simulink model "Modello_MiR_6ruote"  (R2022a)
settings: Solver=VariableStepAuto  StartTime=0.0  StopTime=time_v(end,1)  RelTol=1e-3
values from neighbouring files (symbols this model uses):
  a = 0.250    (= 0.25)    [Modello_MiR_6ruote_script.m]    (also in Modello_MiR_2ruote_script.m; Modello_MiR_6ruote_validato_script.m; Modello_MiR_UR_script.m)
  Att_C = 0.005    [Modello_MiR_6ruote_script.m]
  b = 0.1875    [Modello_MiR_6ruote_script.m]    (also in Modello_MiR_2ruote_script.m; Modello_MiR_6ruote_validato_script.m; Modello_MiR_UR_script.m)
  b_caster = 0.07    [Modello_MiR_6ruote_script.m]    (also in Modello_MiR_2ruote_script.m; Modello_MiR_6ruote_validato_script.m; Modello_MiR_UR_script.m)
  bd = 0.205    [Modello_MiR_6ruote_script.m]    (also in Modello_MiR_2ruote_script.m; Modello_MiR_6ruote_validato_script.m; Modello_MiR_UR_script.m)
  F23fun = @(u) (mv*9.801/4)-u(7)    [Modello_MiR_6ruote_script.m]    (also in Modello_MiR_6ruote_validato_script.m = @(u) (mv*9.801/4)-(mv*h*u(5)+(mv*9.801/4)*(2*a-b_caster*(cos)
  F43fun = @(u) (1/(2*bd))*(mv*u(6)*h+u(7)*(2*bd-b_caster*(sin(u(3))+sin(u(4))))+u(8)*(2*bd-b_caster*(sin(u(1))+sin(u(2)))))    [Modello_MiR_6ruote_script.m]    (also in Modello_MiR_6ruote_validato_script.m = @(u) (1/(2*bd))*(mv*u(6)*h+((mv*h*u(5)+(mv*9.801/4)*(2*a-b_c)
  F63fun = @(u) (mv*h*u(5)+(mv*9.801/4)*(2*a-b_caster*(cos(u(1))+cos(u(2)))))/(4*a-b_caster*(cos(u(1))+cos(u(2)))+b_caster*(cos(u(3))+cos(u(4))))    [Modello_MiR_6ruote_script.m]    (also in Modello_MiR_6ruote_validato_script.m)
  fm_fun = @(u) (u <= -am2 | u >= am2)*0 + (u > -am2 && u <= -am1)*(- u * Mza/(am2 -am1) - Mza * am2/(am2 -am1)) +           + (u > -am1 && u <= am1)*(Mza*u/ am1) + (u > am1 && u < am2)*(Mza * u/(am1 -am2) - Mza * am2/(am1 - am2))    [Modello_MiR_6ruote_script.m]    (also in Modello_MiR_6ruote_validato_script.m = @(u) (u <= -am2 || u >= am2) * 0 + (u > -am2 && u <= -am1) *; Modello_MiR_UR_script.m = @(u) (u <= -am2 || u >= am2) * 0 + (u > -am2 && u <= -am1) *)
  Icw_1 = 1/2 * mcw * rc^2    (= 0.002004225735)    [Modello_MiR_6ruote_script.m]    (also in Modello_MiR_2ruote_script.m; Modello_MiR_6ruote_validato_script.m; Modello_MiR_UR_script.m)
  Icw_2 = 1/12 * mcw * ec^2 + 1/4 * mcw * rc^2    (= 0.00104098243873)    [Modello_MiR_6ruote_script.m]    (also in Modello_MiR_2ruote_script.m; Modello_MiR_6ruote_validato_script.m; Modello_MiR_UR_script.m)
  Idw_1 = 1/2 * mdw * rd^2    (= 0.00551836278784)    [Modello_MiR_6ruote_script.m]    (also in Modello_MiR_2ruote_script.m; Transfer_Function_Gol_Gcl.m = Inertia_vect(jj,1); Modello_MiR_6ruote_validato_script.m; Modello_MiR_UR_script.m)
  iMax = 20.7*1.1    (= 22.77)    [Modello_MiR_6ruote_script.m]    (also in Modello_MiR_2ruote_script.m; Modello_MiR_6ruote_validato_script.m; Modello_MiR_UR_script.m)
  Iv = mv * (l^2 + w^2)  / 12    (= 6.75343333333)    [Modello_MiR_6ruote_script.m]    (also in Modello_MiR_2ruote_script.m; Modello_MiR_6ruote_validato_script.m = 8.95033333333; Modello_MiR_UR_script.m)
  Kc = 0.15    [Modello_MiR_6ruote_script.m]    (also in Modello_MiR_2ruote_script.m; Modello_MiR_6ruote_validato_script.m; Modello_MiR_UR_script.m)
  Ki_i = 1    [Modello_MiR_6ruote_script.m]    (also in Modello_MiR_2ruote_script.m; Modello_MiR_6ruote_validato_script.m; Modello_MiR_UR_script.m)
  Ki_v = 1    [Modello_MiR_6ruote_script.m]    (also in Modello_MiR_2ruote_script.m; Modello_MiR_6ruote_validato_script.m; Modello_MiR_UR_script.m)
  kk = 0.00005    (= 5e-05)    [Modello_MiR_6ruote_script.m]    (also in Modello_MiR_2ruote_script.m; Modello_MiR_6ruote_validato_script.m; Modello_MiR_UR_script.m)
  Kp_i = 5    [Modello_MiR_6ruote_script.m]    (also in Modello_MiR_2ruote_script.m; Modello_MiR_6ruote_validato_script.m; Modello_MiR_UR_script.m)
  Kp_v = 5    [Modello_MiR_6ruote_script.m]    (also in Modello_MiR_2ruote_script.m; Modello_MiR_6ruote_validato_script.m; Modello_MiR_UR_script.m)
  kv = 1.5e-6    (= 1.5e-06)    [Modello_MiR_6ruote_script.m]    (also in Modello_MiR_2ruote_script.m; Modello_MiR_6ruote_validato_script.m; Modello_MiR_UR_script.m)
  L = R * tauE    (= 0.00181134822805)    [Modello_MiR_6ruote_script.m]    (also in Modello_MiR_2ruote_script.m; Modello_MiR_6ruote_validato_script.m; Modello_MiR_UR_script.m)
  mcw = rc^2 * pi * ec * rhopoliu + 1    (= 1.02616357632)    [Modello_MiR_6ruote_script.m]    (also in Modello_MiR_2ruote_script.m; Modello_MiR_6ruote_validato_script.m; Modello_MiR_UR_script.m)
  mv = 83    [Modello_MiR_6ruote_script.m]    (also in Modello_MiR_2ruote_script.m; Modello_MiR_6ruote_validato_script.m = 110; Modello_MiR_UR_script.m)
  Psi_start = pi/2    (= 1.57079632679)    [Modello_MiR_6ruote_script.m]    (also in Modello_MiR_6ruote_validato_script.m = psi_mir(1,1); Modello_MiR_UR_script.m = psi_mir(1,1))
  R = velMax * TorqueMax / (iMax)^2    (= 1.81134822805)    [Modello_MiR_6ruote_script.m]    (also in Modello_MiR_2ruote_script.m; Modello_MiR_6ruote_validato_script.m; Modello_MiR_UR_script.m)
  rap_rid = 10.167    [Modello_MiR_6ruote_script.m]    (also in Modello_MiR_2ruote_script.m; Modello_MiR_6ruote_validato_script.m; Modello_MiR_UR_script.m)
  rc = 0.125/2    (= 0.0625)    [Modello_MiR_6ruote_script.m]    (also in Modello_MiR_2ruote_script.m; Modello_MiR_6ruote_validato_script.m; Modello_MiR_UR_script.m)
  rd = 0.1    [Modello_MiR_6ruote_script.m]    (also in Modello_MiR_2ruote_script.m; Modello_MiR_6ruote_validato_script.m; Modello_MiR_UR_script.m)
  Sx = spline(x ,fl_fun(x),zx)    [Modello_MiR_6ruote_script.m]
  Sy = spline(x ,ft_fun(x),zy)    [Modello_MiR_6ruote_script.m]
  VaMax = Kc * velMax    (= 41.2443991527)    [Modello_MiR_6ruote_script.m]    (also in Modello_MiR_2ruote_script.m; Modello_MiR_6ruote_validato_script.m; Modello_MiR_UR_script.m)
  X_start = input('Inserire coordinata x iniziale')    [Modello_MiR_6ruote_script.m]    (also in Modello_MiR_2ruote_script.m; Modello_MiR_6ruote_validato_script.m = traj(1,1); Modello_MiR_UR_script.m = traj(1,1))
  Y_start = input('Inserire coordinata y iniziale')    [Modello_MiR_6ruote_script.m]    (also in Modello_MiR_2ruote_script.m; Modello_MiR_6ruote_validato_script.m = traj(1,2); Modello_MiR_UR_script.m = traj(1,2))
  zx = linspace(inferior,superi,10001)    [Modello_MiR_6ruote_script.m]
  zy = linspace(inferior,superi,10001)    [Modello_MiR_6ruote_script.m]
libraries: slpidlib x4
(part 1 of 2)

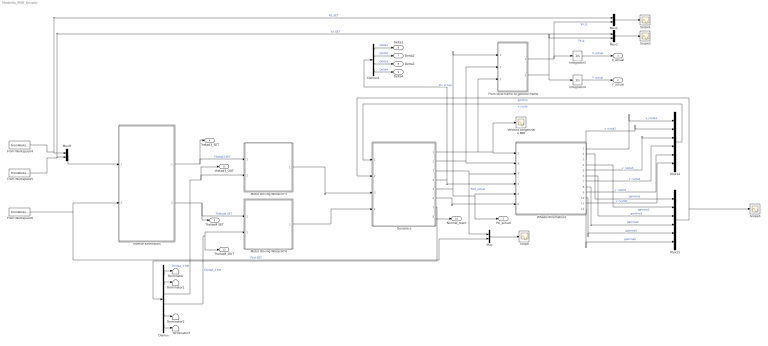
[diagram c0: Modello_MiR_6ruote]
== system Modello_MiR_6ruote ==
  " Wheels Kinematics1" : Subsystem
  Demux : Demux  Outputs=6
  Demux1 : Demux
  Dynamics : Subsystem
  From Workspace4 : FromWorkspace  VariableName=[time_v Xd_set]
  From Workspace5 : FromWorkspace  VariableName=[time_v Yd_set]
  From Workspace6 : FromWorkspace  VariableName=[ time_v psid_set]
  From local frame to general frame : Subsystem
  Integrator3 : Integrator  InitialCondition=X_start
  Integrator4 : Integrator  InitialCondition=Y_start
  Inverse Kinematics : Subsystem
  Motor Driving Wheel N°3 : Subsystem
  Motor Driving Wheel N°4 : Subsystem
  Mux{,1..2,9} (4 alike) : Mux  Inputs=2
  Mux14 : Mux  Inputs=6
  Mux15 : Mux  Inputs=6
  Scope{,1..3} (4 alike) : Scope
  Terminator{,1..3} (4 alike) : Terminator
  Velocità tangenziale MIR : Scope
  Psi_actual : Outport
  Y_actual : Outport  Port=2
  X_actual : Outport  Port=3
  Thetad3_SET : Outport  Port=4
  Thetad4 SET : Outport  Port=5
  Delta1 : Outport  Port=6
  Delta2 : Outport  Port=7
  Delta3 : Outport  Port=8
  Delta4 : Outport  Port=9
  Normal_react : Outport  Port=10
  thetad3_OUT : Outport  Port=11
  Thetad4_OUT : Outport  Port=12
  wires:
  From local frame to general frame/2(Vy_g) -> Mux2/2, Integrator4/1  "Vy_g"
  Mux2/1 -> Scope2/1
  Dynamics/6(Phid) -> " Wheels Kinematics1"/6(Phid)
  " Wheels Kinematics1"/9(v_ruota5) -> Mux14/5  "v_ruota5"
  " Wheels Kinematics1"/4(gamma2) -> Mux15/2  "gamma2"
  " Wheels Kinematics1"/11(v_ruota6) -> Mux14/6  "v_ruota6"
  " Wheels Kinematics1"/12(gamma6) -> Mux15/6  "gamma6"
  " Wheels Kinematics1"/10(gamma5) -> Mux15/5  "gamma5"
  " Wheels Kinematics1"/8(gamma4) -> Mux15/4  "gamma4"
  " Wheels Kinematics1"/3(v_ruota2) -> Mux14/2  "v_ruota2"
  Dynamics/7(Thetad) -> Demux/1
  Motor Driving Wheel N°3/1(Cm_L) -> Dynamics/3(Cm3)
  From Workspace6/1 -> Mux/2, Inverse Kinematics/2(PsiDotSet)  "Psid_SET"
  Mux/1 -> Scope/1
  Dynamics/4(Delta) -> " Wheels Kinematics1"/4(Delta), Demux1/1
  Dynamics/5(Psi) -> From local frame to general frame/1(Psi), " Wheels Kinematics1"/5(Psi), Psi_actual/1  "Psi_actual"
  " Wheels Kinematics1"/7(v_ruota4) -> Mux14/4  "v_ruota4"
  Demux/6 -> Terminator3/1
  Mux15/1 -> Scope3/1, Dynamics/2(gamma)  "gamma"
  " Wheels Kinematics1"/2(gamma1) -> Mux15/1  "gamma1"
  Demux/5 -> Terminator2/1
  Integrator4/1 -> Y_actual/1  "Y_actual"
  Mux9/1 -> Inverse Kinematics/1(vSet)
  Dynamics/1(xd) -> From local frame to general frame/3(Vx), " Wheels Kinematics1"/1(xd), Velocità tangenziale MIR/1
  " Wheels Kinematics1"/5(v_ruota3) -> Mux14/3  "v_ruota3"
  Dynamics/3(Psid) -> " Wheels Kinematics1"/3(Psid), Mux/1  "Psid_actual"
  " Wheels Kinematics1"/6(gamma3) -> Mux15/3  "gamma3"
  Integrator3/1 -> X_actual/1  "X_actual"
  Inverse Kinematics/2(ThetaDotR) -> Thetad4 SET/1, Motor Driving Wheel N°4/1(ThetadR_SET)  "Thetad4 SET"
  Demux/4 -> Thetad4_OUT/1, Motor Driving Wheel N°4/2(ThetadR_FB)  "Thetad_4 F/B"
  Demux/2 -> Terminator1/1
  From local frame to general frame/1(Vx_g) -> Mux1/2, Integrator3/1  "Vx_g"
  Mux14/1 -> Dynamics/1(v_ruote)  "v_ruote"
  Dynamics/2(yd) -> From local frame to general frame/2(Vy), " Wheels Kinematics1"/2(yd)
  Demux/1 -> Terminator/1
  " Wheels Kinematics1"/1(v_ruota1) -> Mux14/1  "v_ruota1"
  Inverse Kinematics/1(ThetaDotL) -> Thetad3_SET/1, Motor Driving Wheel N°3/1(ThetadL_SET)  "Thetad3 SET"
  Mux1/1 -> Scope1/1
  From Workspace5/1 -> Mux2/1, Mux9/2  "Yd_SET"
  Motor Driving Wheel N°4/1(Cm_R) -> Dynamics/4(Cm4)
  Demux/3 -> thetad3_OUT/1, Motor Driving Wheel N°3/2(ThetadL_FB)  "Thetad_3 F/B"
  From Workspace4/1 -> Mux1/1, Mux9/1  "Xd_SET"
  Demux1/1 -> Delta1/1  "Delta1"
  Demux1/2 -> Delta2/1  "Delta2"
  Demux1/3 -> Delta3/1  "Delta3"
  Demux1/4 -> Delta4/1  "Delta4"
  Dynamics/8(Normal_react) -> Normal_react/1

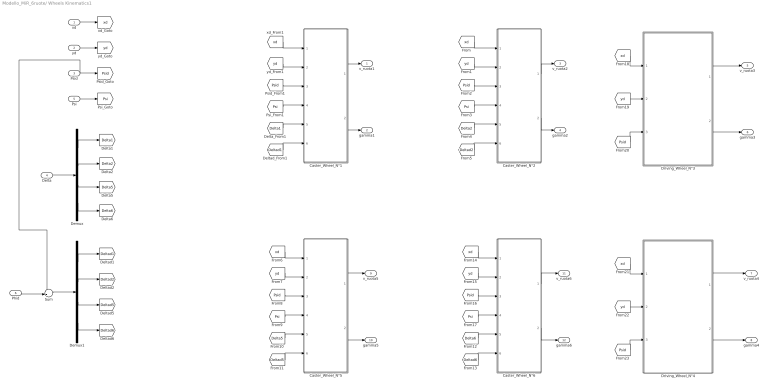
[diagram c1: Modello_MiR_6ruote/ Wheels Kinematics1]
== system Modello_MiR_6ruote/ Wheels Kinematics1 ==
  xd : Inport
  yd : Inport  Port=2
  Psid : Inport  Port=3
  Delta : Inport  Port=4
  Psi : Inport  Port=5
  Phid : Inport  Port=6
  Caster_Wheel_N°1 : Subsystem
  Caster_Wheel_N°2 : Subsystem
  Caster_Wheel_N°5 : Subsystem
  Caster_Wheel_N°6 : Subsystem
  Demux : Demux
  Demux1 : Demux
  Driving_Wheel_N°3 : Subsystem
  Driving_Wheel_N°4 : Subsystem
  Sum : Sum  Inputs=-+|
  v_ruota1 : Outport  PortDimensions=1
  gamma1 : Outport  Port=2  PortDimensions=1
  v_ruota2 : Outport  Port=3  PortDimensions=1
  gamma2 : Outport  Port=4  PortDimensions=1
  v_ruota3 : Outport  Port=5  PortDimensions=1
  gamma3 : Outport  Port=6  PortDimensions=1
  v_ruota4 : Outport  Port=7  PortDimensions=1
  gamma4 : Outport  Port=8  PortDimensions=1
  v_ruota5 : Outport  Port=9  PortDimensions=1
  gamma5 : Outport  Port=10  PortDimensions=1
  v_ruota6 : Outport  Port=11  PortDimensions=1
  gamma6 : Outport  Port=12  PortDimensions=1
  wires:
  xd/1 -> [xd]
  yd/1 -> [yd]
  Psid/1 -> [Psid], Sum/1
  Delta/1 -> Demux/1
  Demux/1 -> [Delta1]
  Demux/2 -> [Delta2]
  Demux/3 -> [Delta5]
  Demux/4 -> [Delta6]
  Psi/1 -> [Psi]
  Phid/1 -> Sum/2
  Demux1/1 -> [Deltad1]
  Demux1/2 -> [Deltad2]
  Demux1/3 -> [Deltad5]
  Demux1/4 -> [Deltad6]
  [xd] -> Caster_Wheel_N°1/1(xd_From1)
  [yd] -> Caster_Wheel_N°1/2(yd_From1)
  [Psid] -> Caster_Wheel_N°1/3(Psid_From1)
  [Psi] -> Caster_Wheel_N°1/4(Psi_From1)
  [Delta1] -> Caster_Wheel_N°1/5(Delta_From1)
  [Deltad1] -> Caster_Wheel_N°1/6(Deltad_From1)
  Caster_Wheel_N°1/1(v_ruota1) -> v_ruota1/1
  Caster_Wheel_N°1/2(gamma1) -> gamma1/1
  [yd] -> Caster_Wheel_N°2/2(yd_From1)
  [Psi] -> Caster_Wheel_N°2/4(Psi_From1)
  [Psid] -> Caster_Wheel_N°2/3(Psid_From1)
  [xd] -> Caster_Wheel_N°2/1(xd_From1)
  [Deltad2] -> Caster_Wheel_N°2/6(Deltad_From2)
  Caster_Wheel_N°2/2(gamma2) -> gamma2/1
  [Delta2] -> Caster_Wheel_N°2/5(Delta_From2)
  Caster_Wheel_N°2/1(v_ruota2) -> v_ruota2/1
  [xd] -> Caster_Wheel_N°5/1(xd_From1)
  Caster_Wheel_N°5/2(gamma5) -> gamma5/1
  Caster_Wheel_N°5/1(v_ruota5) -> v_ruota5/1
  [Psid] -> Caster_Wheel_N°5/3(Psid_From1)
  [Deltad5] -> Caster_Wheel_N°5/6(Deltad_From5)
  [yd] -> Caster_Wheel_N°5/2(yd_From1)
  [Delta5] -> Caster_Wheel_N°5/5(Delta_From5)
  [Psi] -> Caster_Wheel_N°5/4(Psi_From1)
  Caster_Wheel_N°6/1(v_ruota6) -> v_ruota6/1
  [yd] -> Caster_Wheel_N°6/2(yd_From1)
  [Psid] -> Caster_Wheel_N°6/3(Psid_From1)
  [Psi] -> Caster_Wheel_N°6/4(Psi_From1)
  Caster_Wheel_N°6/2(gamma6) -> gamma6/1
  [xd] -> Caster_Wheel_N°6/1(xd_From1)
  [Delta6] -> Caster_Wheel_N°6/5(Delta_From6)
  [Deltad6] -> Caster_Wheel_N°6/6(Deltad_From6)
  [xd] -> Driving_Wheel_N°3/1(xd_From1)
  [yd] -> Driving_Wheel_N°3/2(yd_From1)
  [Psid] -> Driving_Wheel_N°3/3(Psid_From1)
  [xd] -> Driving_Wheel_N°4/1(xd_From1)
  [yd] -> Driving_Wheel_N°4/2(yd_From1)
  [Psid] -> Driving_Wheel_N°4/3(Psid_From1)
  Driving_Wheel_N°3/1(v_ruota3) -> v_ruota3/1
  Driving_Wheel_N°3/2(gamma3) -> gamma3/1
  Driving_Wheel_N°4/1(v_ruota4) -> v_ruota4/1
  Driving_Wheel_N°4/2(gamma4) -> gamma4/1
  Sum/1 -> Demux1/1

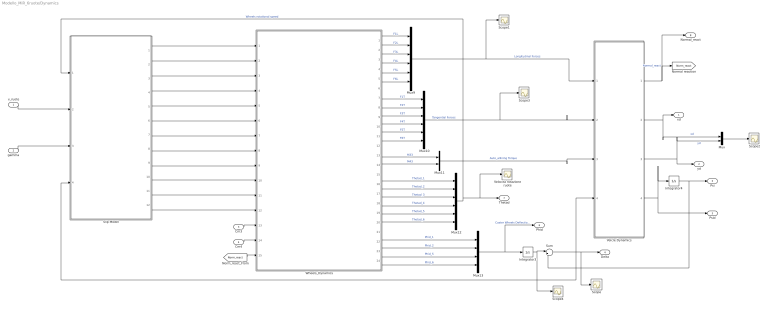
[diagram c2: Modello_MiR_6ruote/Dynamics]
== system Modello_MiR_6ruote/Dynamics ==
  v_ruote : Inport
  gamma : Inport  Port=2
  Cm3 : Inport  Port=3
  Cm4 : Inport  Port=4
  Integrator3 : Integrator  InitialCondition=Psi_start
  Integrator4 : Integrator  InitialCondition=Psi_start
  Mux : Mux  Inputs=2
  Mux10 : Mux  Inputs=6
  Mux11 : Mux  Inputs=2
  Mux12 : Mux  Inputs=6
  Mux13 : Mux
  Mux9 : Mux  Inputs=6
  Scope{,1..4} (5 alike) : Scope
  Slip Model : Subsystem
  Sum : Sum  Inputs=|+-
  Veicle Dynamics : Subsystem
  Velocità rotazione ruote : Scope
  Wheels_Dynamics : Subsystem
  xd : Outport
  yd : Outport  Port=2
  Psid : Outport  Port=3
  Delta : Outport  Port=4
  Psi : Outport  Port=5
  Phid : Outport  Port=6
  Thetad : Outport  Port=7
  Normal_react : Outport  Port=8
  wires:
  Wheels_Dynamics/14(M43) -> Mux11/2  "M43"
  Wheels_Dynamics/23(Phid_5) -> Mux13/3  "Phid_5"
  Wheels_Dynamics/8(F2T) -> Mux10/2  "F2T"
  Wheels_Dynamics/12(F6T) -> Mux10/6  "F6T"
  Wheels_Dynamics/19(Thetad_5) -> Mux12/5  "Thetad_5"
  Wheels_Dynamics/18(Thetad_4) -> Mux12/4  "Thetad_4"
  Slip Model/1(Sigma1) -> Wheels_Dynamics/1(Sigma1)
  Wheels_Dynamics/2(F2L) -> Mux9/2  "F2L"
  Wheels_Dynamics/4(F4L) -> Mux9/4  "F4L"
  Wheels_Dynamics/3(F3L) -> Mux9/3  "F3L"
  Veicle Dynamics/4(Psid) -> Psid/1, Integrator4/1
  Wheels_Dynamics/1(F1L) -> Mux9/1  "F1L"
  Slip Model/3(Sigma3) -> Wheels_Dynamics/3(Sigma3)
  Slip Model/11(alpha5) -> Wheels_Dynamics/11(alpha5)
  Wheels_Dynamics/5(F5L) -> Mux9/5  "F5L"
  Slip Model/9(alpha3) -> Wheels_Dynamics/9(alpha3)
  Wheels_Dynamics/16(Thetad_2) -> Mux12/2  "Thetad_2"
  Mux13/1 -> Integrator3/1, Phid/1  "Caster Wheels Deflection Velocity"
  Cm3/1 -> Wheels_Dynamics/13(Cm3)
  Mux11/1 -> Veicle Dynamics/3(M)  "Auto_allining Torque"
  Wheels_Dynamics/10(F4T) -> Mux10/4  "F4T"
  Wheels_Dynamics/13(M33) -> Mux11/1  "M33"
  Mux12/1 -> Slip Model/1(Thetad_ruote), Velocità rotazione ruote/1, Thetad/1  "Wheels rotational speed"
  Mux10/1 -> Scope3/1, Veicle Dynamics/2(FT)  "Tangential Forces"
  Slip Model/5(Sigma5) -> Wheels_Dynamics/5(Sigma5)
  Wheels_Dynamics/21(Phid_1) -> Mux13/1  "Phid_1"
  Wheels_Dynamics/6(F6L) -> Mux9/6  "F6L"
  Wheels_Dynamics/17(Thetad_3) -> Mux12/3  "Thetad_3"
  Wheels_Dynamics/15(Thetad_1) -> Mux12/1  "Thetad_1"
  Wheels_Dynamics/24(Phid_6) -> Mux13/4  "Phid_6"
  Wheels_Dynamics/11(F5T) -> Mux10/5  "F5T"
  Wheels_Dynamics/9(F3T) -> Mux10/3  "F3T"
  Wheels_Dynamics/7(F1T) -> Mux10/1  "F1T"
  Wheels_Dynamics/22(Phid_2) -> Mux13/2  "Phid_2"
  Veicle Dynamics/1(Normal_react) -> Normal_react/1, [Norm_react]  "Normal_react"
  Veicle Dynamics/2(xd) -> Mux/1, xd/1  "xd"
  Integrator3/1 -> Scope4/1, Sum/1
  Wheels_Dynamics/20(Thetad_6) -> Mux12/6  "Thetad_6"
  Slip Model/8(alpha2) -> Wheels_Dynamics/8(alpha2)
  Integrator4/1 -> Sum/2, Psi/1
  [Norm_react] -> Wheels_Dynamics/15(Normal_React)
  Veicle Dynamics/3(yd) -> Mux/2, yd/1  "yd"
  Mux9/1 -> Scope1/1, Veicle Dynamics/1(FL)  "Longitudinal Forces"
  Slip Model/4(Sigma4) -> Wheels_Dynamics/4(Sigma4)
  Slip Model/10(alpha4) -> Wheels_Dynamics/10(alpha4)
  Slip Model/12(alpha6) -> Wheels_Dynamics/12(alpha6)
  Slip Model/7(alpha1) -> Wheels_Dynamics/7(alpha1)
  Slip Model/2(Sigma2) -> Wheels_Dynamics/2(Sigma2)
  Slip Model/6(Sigma6) -> Wheels_Dynamics/6(Sigma6)
  v_ruote/1 -> Slip Model/2(v_ruote)
  gamma/1 -> Slip Model/3(gamma)
  Cm4/1 -> Wheels_Dynamics/14(Cm4)
  Mux/1 -> Scope2/1
  Sum/1 -> Slip Model/4(Delta), Scope/1, Delta/1, Veicle Dynamics/4(Delta)

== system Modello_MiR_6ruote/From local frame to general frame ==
  Psi : Inport
  Vy : Inport  Port=2
  Vx : Inport  Port=3
  Cos : Trigonometry  Operator=cos
  Product{,1..3} (4 alike) : Product
  Sin : Trigonometry
  Sum : Sum  Inputs=-+
  Sum1 : Sum  Inputs=|++
  Vx_g : Outport
  Vy_g : Outport  Port=2
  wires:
  Product/1 -> Sum/2
  Sin/1 -> Product2/2, Product1/2
  Product1/1 -> Sum/1
  Vx/1 -> Product2/1, Product/1
  Product2/1 -> Sum1/1
  Cos/1 -> Product3/1, Product/2
  Product3/1 -> Sum1/2
  Psi/1 -> Sin/1, Cos/1
  Vy/1 -> Product3/2, Product1/1
  Sum/1 -> Vx_g/1
  Sum1/1 -> Vy_g/1

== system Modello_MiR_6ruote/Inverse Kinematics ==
  vSet : Inport
  PsiDotSet : Inport  Port=2
  Demux : Demux  Outputs=2
  Integrator : Integrator  InitialCondition=Psi_start
  MATLAB Function : MATLAB Function  TreatAsAtomicUnit=on
  MATLAB Function1 : MATLAB Function  TreatAsAtomicUnit=on
  Scope1 : Scope
  Scope2 : Scope
  ThetaDotL : Outport
  ThetaDotR : Outport  Port=2
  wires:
  vSet/1 -> Demux/1
  Demux/1 -> MATLAB Function1/2(Xd_set), MATLAB Function/2(Xd_set)  "Xd_set"
  Demux/2 -> MATLAB Function1/3(Yd_set), MATLAB Function/3(Yd_set)  "Yd_set"
  PsiDotSet/1 -> MATLAB Function1/4(psid_set), MATLAB Function/4(psid_set), Integrator/1
  Integrator/1 -> MATLAB Function1/1(psi_set), MATLAB Function/1(psi_set)  "Psi_set"
  MATLAB Function/1(Thetad_DR_SET) -> Scope1/1, ThetaDotR/1
  MATLAB Function1/1(Thetad_DL_SET) -> Scope2/1, ThetaDotL/1

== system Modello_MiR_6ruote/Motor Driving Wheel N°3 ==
  ThetadL_SET : Inport
  ThetadL_FB : Inport  Port=2
  Gain : Gain  Gain=rap_rid
  Gain1 : Gain  Gain=rap_rid
  Subsystem : Subsystem
  Subsystem1 : Subsystem
  Cm_L : Outport  PortDimensions=1
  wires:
  Subsystem/1(VaRif) -> Subsystem1/1(VaRif)
  Subsystem1/2(iFB) -> Subsystem/3(iFB)
  ThetadL_SET/1 -> Gain1/1
  ThetadL_FB/1 -> Gain/1
  Subsystem1/1(Torque Cm) -> Cm_L/1
  Gain/1 -> Subsystem1/2(Thetad_FB), Subsystem/2(Thetad_FB)
  Gain1/1 -> Subsystem/1(Thetad_SET)

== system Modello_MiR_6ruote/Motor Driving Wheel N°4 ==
  ThetadR_SET : Inport
  ThetadR_FB : Inport  Port=2
  Gain : Gain  Gain=rap_rid
  Gain1 : Gain  Gain=rap_rid
  Subsystem : Subsystem
  Subsystem1 : Subsystem
  Cm_R : Outport  PortDimensions=1
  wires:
  Subsystem1/2(iFB) -> Subsystem/3(iFB)
  ThetadR_SET/1 -> Gain1/1
  Subsystem/1(VaRif) -> Subsystem1/1(VaRif)
  ThetadR_FB/1 -> Gain/1
  Subsystem1/1(Torque Cm) -> Cm_R/1
  Gain/1 -> Subsystem1/2(Thetad_FB), Subsystem/2(Thetad_FB)
  Gain1/1 -> Subsystem/1(Thetad_SET)

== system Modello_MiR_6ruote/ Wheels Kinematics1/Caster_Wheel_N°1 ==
  xd_From1 : Inport
  yd_From1 : Inport  Port=2
  Psid_From1 : Inport  Port=3
  Psi_From1 : Inport  Port=4
  Delta_From1 : Inport  Port=5
  Deltad_From1 : Inport  Port=6
  Interpreted MATLAB Function : MATLABFcn  MATLABFcn=(u(1)^2+u(2)^2)^0.5
  Interpreted MATLAB Function2 : MATLABFcn  MATLABFcn=asin(u(2)/((u(1)^2+u(2)^2)^0.5+1*(((u(1)^2+u(2)^2)^0.5)==0)))
  Mux : Mux  Inputs=6
  Mux1 : Mux  Inputs=2
  xd_ruota1 : MATLABFcn  MATLABFcn=(u(6)+u(3))*b_caster*sin(u(5))+u(1)-u(3)*b
  yd_ruota1 : MATLABFcn  MATLABFcn=-(u(6)+u(3))*b_caster*cos(u(5))+u(2)+u(3)*a
  v_ruota1 : Outport
  gamma1 : Outport  Port=2
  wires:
  Mux/1 -> xd_ruota1/1, yd_ruota1/1
  Mux1/1 -> Interpreted MATLAB Function/1, Interpreted MATLAB Function2/1
  yd_ruota1/1 -> Mux1/2  "yd_ruota1"
  yd_From1/1 -> Mux/2
  xd_ruota1/1 -> Mux1/1  "xd_ruota1"
  xd_From1/1 -> Mux/1
  Psid_From1/1 -> Mux/3
  Delta_From1/1 -> Mux/5
  Psi_From1/1 -> Mux/4
  Deltad_From1/1 -> Mux/6
  Interpreted MATLAB Function2/1 -> gamma1/1  "gamma1"
  Interpreted MATLAB Function/1 -> v_ruota1/1  "v_ruota1"

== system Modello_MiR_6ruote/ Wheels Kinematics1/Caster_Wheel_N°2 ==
  xd_From1 : Inport
  yd_From1 : Inport  Port=2
  Psid_From1 : Inport  Port=3
  Psi_From1 : Inport  Port=4
  Delta_From2 : Inport  Port=5
  Deltad_From2 : Inport  Port=6
  Interpreted MATLAB Function : MATLABFcn  MATLABFcn=(u(1)^2+u(2)^2)^0.5
  Interpreted MATLAB Function2 : MATLABFcn  MATLABFcn=asin(u(2)/((u(1)^2+u(2)^2)^0.5+1*(((u(1)^2+u(2)^2)^0.5)==0)))
  Mux : Mux  Inputs=6
  Mux1 : Mux  Inputs=2
  xd_ruota2 : MATLABFcn  MATLABFcn=(u(6)+u(3))*b_caster*sin(u(5))+u(1)+u(3)*b
  yd_ruota2 : MATLABFcn  MATLABFcn=-(u(6)+u(3))*b_caster*cos(u(5))+u(2)+u(3)*a
  v_ruota2 : Outport
  gamma2 : Outport  Port=2
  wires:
  Mux/1 -> xd_ruota2/1, yd_ruota2/1
  Mux1/1 -> Interpreted MATLAB Function/1, Interpreted MATLAB Function2/1
  yd_ruota2/1 -> Mux1/2  "yd_ruota2"
  yd_From1/1 -> Mux/2
  xd_ruota2/1 -> Mux1/1  "xd_ruota2"
  xd_From1/1 -> Mux/1
  Psid_From1/1 -> Mux/3
  Delta_From2/1 -> Mux/5
  Psi_From1/1 -> Mux/4
  Deltad_From2/1 -> Mux/6
  Interpreted MATLAB Function2/1 -> gamma2/1  "gamma2"
  Interpreted MATLAB Function/1 -> v_ruota2/1  "v_ruota2"

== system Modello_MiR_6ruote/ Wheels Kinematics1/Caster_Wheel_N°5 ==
  xd_From1 : Inport
  yd_From1 : Inport  Port=2
  Psid_From1 : Inport  Port=3
  Psi_From1 : Inport  Port=4
  Delta_From5 : Inport  Port=5
  Deltad_From5 : Inport  Port=6
  Interpreted MATLAB Function : MATLABFcn  MATLABFcn=(u(1)^2+u(2)^2)^0.5
  Interpreted MATLAB Function2 : MATLABFcn  MATLABFcn=asin(u(2)/((u(1)^2+u(2)^2)^0.5+1*(((u(1)^2+u(2)^2)^0.5)==0)))
  Mux : Mux  Inputs=6
  Mux1 : Mux  Inputs=2
  xd_ruota5 : MATLABFcn  MATLABFcn=(u(6)+u(3))*b_caster*sin(u(5))+u(1)-u(3)*a
  yd_ruota5 : MATLABFcn  MATLABFcn=-(u(6)+u(3))*b_caster*cos(u(5))+u(2)-u(3)*b
  v_ruota5 : Outport
  gamma5 : Outport  Port=2
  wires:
  Mux/1 -> xd_ruota5/1, yd_ruota5/1
  Mux1/1 -> Interpreted MATLAB Function/1, Interpreted MATLAB Function2/1
  yd_ruota5/1 -> Mux1/2  "yd_ruota5"
  yd_From1/1 -> Mux/2
  xd_ruota5/1 -> Mux1/1  "xd_ruota5"
  xd_From1/1 -> Mux/1
  Psid_From1/1 -> Mux/3
  Delta_From5/1 -> Mux/5
  Psi_From1/1 -> Mux/4
  Deltad_From5/1 -> Mux/6
  Interpreted MATLAB Function2/1 -> gamma5/1  "gamma5"
  Interpreted MATLAB Function/1 -> v_ruota5/1  "v_ruota5"

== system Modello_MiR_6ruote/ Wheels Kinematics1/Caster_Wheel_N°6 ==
  xd_From1 : Inport
  yd_From1 : Inport  Port=2
  Psid_From1 : Inport  Port=3
  Psi_From1 : Inport  Port=4
  Delta_From6 : Inport  Port=5
  Deltad_From6 : Inport  Port=6
  Interpreted MATLAB Function : MATLABFcn  MATLABFcn=(u(1)^2+u(2)^2)^0.5
  Interpreted MATLAB Function2 : MATLABFcn  MATLABFcn=asin(u(2)/((u(1)^2+u(2)^2)^0.5+1*(((u(1)^2+u(2)^2)^0.5)==0)))
  Mux : Mux  Inputs=6
  Mux1 : Mux  Inputs=2
  xd_ruota6 : MATLABFcn  MATLABFcn=(u(6)+u(3))*b_caster*sin(u(5))+u(1)+u(3)*b
  yd_ruota6 : MATLABFcn  MATLABFcn=-(u(6)+u(3))*b_caster*cos(u(5))+u(2)-u(3)*a
  v_ruota6 : Outport
  gamma6 : Outport  Port=2
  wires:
  Mux/1 -> xd_ruota6/1, yd_ruota6/1
  Mux1/1 -> Interpreted MATLAB Function/1, Interpreted MATLAB Function2/1
  yd_ruota6/1 -> Mux1/2  "yd_ruota6"
  yd_From1/1 -> Mux/2
  xd_ruota6/1 -> Mux1/1  "xd_ruota6"
  xd_From1/1 -> Mux/1
  Psid_From1/1 -> Mux/3
  Delta_From6/1 -> Mux/5
  Psi_From1/1 -> Mux/4
  Deltad_From6/1 -> Mux/6
  Interpreted MATLAB Function2/1 -> gamma6/1  "gamma6"
  Interpreted MATLAB Function/1 -> v_ruota6/1  "v_ruota6"

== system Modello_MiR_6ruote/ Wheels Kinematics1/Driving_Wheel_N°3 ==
  xd_From1 : Inport
  yd_From1 : Inport  Port=2
  Psid_From1 : Inport  Port=3
  Interpreted MATLAB Function : MATLABFcn  MATLABFcn=u(1) - u(3)*bd
  Interpreted MATLAB Function1 : MATLABFcn  MATLABFcn=u(2)
  Interpreted MATLAB Function3 : MATLABFcn  MATLABFcn=asin(u(2)/((u(1)^2+u(2)^2)^0.5+1*(((u(1)^2+u(2)^2)^0.5)==0)))
  Mux : Mux  Inputs=3
  Mux1 : Mux  Inputs=2
  Scope : Scope
  v_ruota3 : Outport
  gamma3 : Outport  Port=2
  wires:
  yd_From1/1 -> Mux/2
  xd_From1/1 -> Mux/1
  Psid_From1/1 -> Mux/3
  Mux/1 -> Interpreted MATLAB Function1/1, Interpreted MATLAB Function/1
  Interpreted MATLAB Function1/1 -> Mux1/2  "yd_ruota3"
  Interpreted MATLAB Function3/1 -> gamma3/1  "gamma3"
  Mux1/1 -> Interpreted MATLAB Function3/1
  Interpreted MATLAB Function/1 -> v_ruota3/1, Mux1/1, Scope/1  "v_ruota3"

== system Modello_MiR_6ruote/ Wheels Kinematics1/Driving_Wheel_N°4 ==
  xd_From1 : Inport
  yd_From1 : Inport  Port=2
  Psid_From1 : Inport  Port=3
  Interpreted MATLAB Function : MATLABFcn  MATLABFcn=u(1) + u(3)*bd
  Interpreted MATLAB Function1 : MATLABFcn  MATLABFcn=u(2)
  Interpreted MATLAB Function3 : MATLABFcn  MATLABFcn=asin(u(2)/((u(1)^2+u(2)^2)^0.5+1*(((u(1)^2+u(2)^2)^0.5)==0)))
  Mux : Mux  Inputs=3
  Mux1 : Mux  Inputs=2
  Scope : Scope
  v_ruota4 : Outport
  gamma4 : Outport  Port=2
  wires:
  yd_From1/1 -> Mux/2
  xd_From1/1 -> Mux/1
  Psid_From1/1 -> Mux/3
  Mux/1 -> Interpreted MATLAB Function1/1, Interpreted MATLAB Function/1
  Interpreted MATLAB Function1/1 -> Mux1/2  "yd_ruota4"
  Mux1/1 -> Interpreted MATLAB Function3/1
  Interpreted MATLAB Function/1 -> v_ruota4/1, Mux1/1, Scope/1  "v_ruota4"
  Interpreted MATLAB Function3/1 -> gamma4/1  "gamma4"

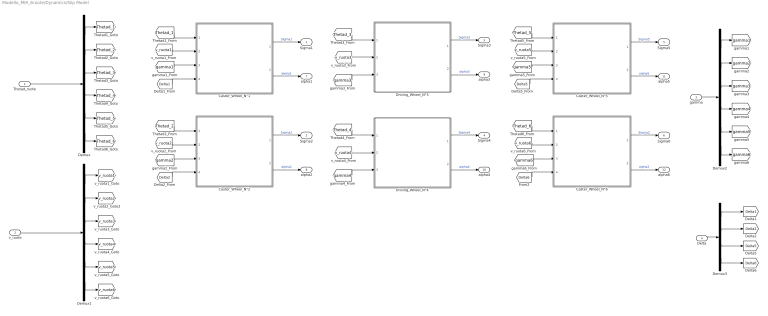
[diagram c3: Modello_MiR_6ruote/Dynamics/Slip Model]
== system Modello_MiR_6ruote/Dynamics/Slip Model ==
  Thetad_ruote : Inport
  v_ruote : Inport  Port=2
  gamma : Inport  Port=3
  Delta : Inport  Port=4
  Caster_Wheel_N°1 : Subsystem
  Caster_Wheel_N°2 : Subsystem
  Caster_Wheel_N°5 : Subsystem
  Caster_Wheel_N°6 : Subsystem
  Demux : Demux  Outputs=6
  Demux1 : Demux  Outputs=6
  Demux2 : Demux  Outputs=6
  Demux3 : Demux
  Driving_Wheel_N°3 : Subsystem
  Driving_Wheel_N°4 : Subsystem
  Sigma1 : Outport  PortDimensions=1
  Sigma2 : Outport  Port=2  PortDimensions=1
  Sigma3 : Outport  Port=3  PortDimensions=1
  Sigma4 : Outport  Port=4  PortDimensions=1
  Sigma5 : Outport  Port=5  PortDimensions=1
  Sigma6 : Outport  Port=6  PortDimensions=1
  alpha1 : Outport  Port=7  PortDimensions=1
  alpha2 : Outport  Port=8  PortDimensions=1
  alpha3 : Outport  Port=9  PortDimensions=1
  alpha4 : Outport  Port=10  PortDimensions=1
  alpha5 : Outport  Port=11  PortDimensions=1
  alpha6 : Outport  Port=12  PortDimensions=1
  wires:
  Caster_Wheel_N°1/2(alpha1) -> alpha1/1  "alpha1"
  Demux/3 -> [Thetad_3]
  [Delta5] -> Caster_Wheel_N°5/4(Delta5)
  Demux1/1 -> [v_ruota1]
  Driving_Wheel_N°3/2(alpha3) -> alpha3/1  "alpha3"
  Demux1/6 -> [v_ruota6]
  Caster_Wheel_N°5/2(alpha5) -> alpha5/1  "alpha5"
  Demux1/2 -> [v_ruota2]
  Demux/1 -> [Thetad_1]
  Demux3/2 -> [Delta2]
  [v_ruota6] -> Caster_Wheel_N°6/2(v_ruota6)
  Driving_Wheel_N°4/1(Sigma4) -> Sigma4/1  "Sigma4"
  Demux2/5 -> [gamma5]
  Caster_Wheel_N°6/2(alpha6) -> alpha6/1  "alpha2"
  Driving_Wheel_N°3/1(Sigma3) -> Sigma3/1  "Sigma3"
  [Thetad_1] -> Caster_Wheel_N°1/1(Thetad_1)
  Demux/2 -> [Thetad_2]
  Driving_Wheel_N°4/2(alpha4) -> alpha4/1  "alpha4"
  Demux1/4 -> [v_ruota4]
  Thetad_ruote/1 -> Demux/1
  [gamma6] -> Caster_Wheel_N°6/3(gamma6)
  Caster_Wheel_N°2/2(alpha2) -> alpha2/1  "alpha2"
  Caster_Wheel_N°5/1(Sigma5) -> Sigma5/1  "Sigma5"
  [v_ruota3] -> Driving_Wheel_N°3/2(v_ruota3)
  Caster_Wheel_N°1/1(Sigma1) -> Sigma1/1  "Sigma1"
  [Thetad_4] -> Driving_Wheel_N°4/1(Thetad_4)
  Demux/5 -> [Thetad_5]
  Caster_Wheel_N°2/1(Sigma2) -> Sigma2/1  "Sigma2"
  [gamma1] -> Caster_Wheel_N°1/3(gamma1)
  Demux/4 -> [Thetad_4]
  [v_ruota4] -> Driving_Wheel_N°4/2(v_ruota4)
  Demux3/1 -> [Delta1]
  Caster_Wheel_N°6/1(Sigma6) -> Sigma6/1  "Sigma2"
  Demux3/3 -> [Delta5]
  Demux/6 -> [Thetad_6]
  Demux2/6 -> [gamma6]
  [Thetad_5] -> Caster_Wheel_N°5/1(Thetad_5)
  [Delta1] -> Caster_Wheel_N°1/4(Delta1)
  Demux1/5 -> [v_ruota5]
  Delta/1 -> Demux3/1
  gamma/1 -> Demux2/1
  [Thetad_3] -> Driving_Wheel_N°3/1(Thetad_3)
  v_ruote/1 -> Demux1/1
  Demux2/4 -> [gamma4]
  Demux2/1 -> [gamma1]
  Demux2/2 -> [gamma2]
  [v_ruota2] -> Caster_Wheel_N°2/2(v_ruota2)
  [gamma5] -> Caster_Wheel_N°5/3(gamma5)
  Demux2/3 -> [gamma3]
  [gamma4] -> Driving_Wheel_N°4/3(gamma4)
  [Thetad_2] -> Caster_Wheel_N°2/1(Thetad_2)
  [v_ruota1] -> Caster_Wheel_N°1/2(v_ruota1)
  [gamma2] -> Caster_Wheel_N°2/3(gamma2)
  Demux1/3 -> [v_ruota3]
  [Delta6] -> Caster_Wheel_N°6/4(Delta6)
  [Thetad_6] -> Caster_Wheel_N°6/1(Thetad_6)
  Demux3/4 -> [Delta6]
  [Delta2] -> Caster_Wheel_N°2/4(Delta2)
  [gamma3] -> Driving_Wheel_N°3/3(gamma3)
  [v_ruota5] -> Caster_Wheel_N°5/2(v_ruota5)

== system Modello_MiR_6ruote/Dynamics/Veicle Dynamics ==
  FL : Inport
  FT : Inport  Port=2
  M : Inport  Port=3
  Delta : Inport  Port=4
  Demux : Demux
  Integrator : Integrator
  Integrator1 : Integrator
  Integrator6 : Integrator
  Mux14 : Mux  Inputs=6
  Normal Reaction : Subsystem
  Rotation Dynamics : Subsystem
  Rotational Matrix : MATLAB Function  TreatAsAtomicUnit=on
  Scope : Scope
  Translation Dynamics : Subsystem
  Normal_react : Outport
  xd : Outport  Port=2  PortDimensions=1
  yd : Outport  Port=3  PortDimensions=1
  Psid : Outport  Port=4  PortDimensions=1
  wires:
  Normal Reaction/4(F43) -> Mux14/4  "F43"
  Demux/1 -> Normal Reaction/1(Delta1)
  Demux/2 -> Normal Reaction/2(Delta2)
  Normal Reaction/5(F53) -> Mux14/5  "F53"
  Demux/4 -> Normal Reaction/4(Delta6)
  Normal Reaction/1(F13) -> Mux14/1  "F13"
  Rotation Dynamics/1(Psidd) -> Integrator6/1
  Normal Reaction/2(F23) -> Mux14/2  "F23"
  Normal Reaction/6(F63) -> Mux14/6  "F63"
  Demux/3 -> Normal Reaction/3(Delta5)
  Normal Reaction/3(F33) -> Mux14/3  "F33"
  Integrator6/1 -> Psid/1, Translation Dynamics/5(Psid)  "Psid"
  Mux14/1 -> Scope/1, Normal_react/1
  Delta/1 -> Rotation Dynamics/2("Delta "), Demux/1, Rotational Matrix/3(Delta)
  Rotational Matrix/2(Fy_generalized) -> Rotation Dynamics/3(Fy_generalized), Translation Dynamics/2(Fy_generalized)
  FL/1 -> Rotational Matrix/1(FL)
  FT/1 -> Rotational Matrix/2(FT)
  Rotational Matrix/1(Fx_generalized) -> Rotation Dynamics/1(Fx_generalized), Translation Dynamics/1(Fx_generalized)
  Translation Dynamics/1(xdd) -> Integrator/1
  Translation Dynamics/2(ydd) -> Integrator1/1
  Integrator/1 -> Translation Dynamics/3(xd), xd/1
  Integrator1/1 -> Translation Dynamics/4(yd), yd/1
  M/1 -> Rotation Dynamics/4(M)
  Translation Dynamics/3(a_tau) -> Normal Reaction/5(a_tau)
  Translation Dynamics/4(a_n) -> Normal Reaction/6(a_n)

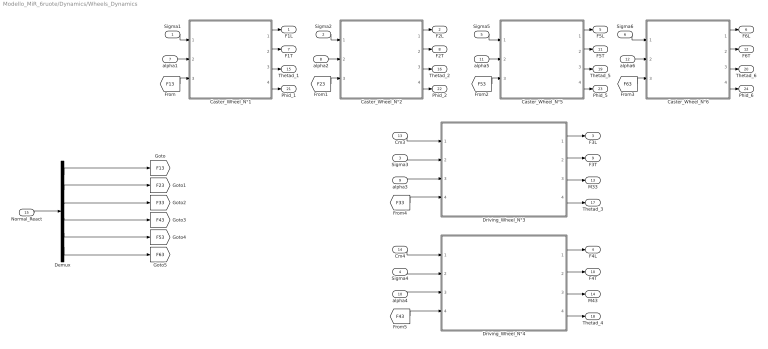
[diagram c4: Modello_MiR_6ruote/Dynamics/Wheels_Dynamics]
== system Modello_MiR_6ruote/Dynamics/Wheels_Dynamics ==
  Sigma1 : Inport
  Sigma2 : Inport  Port=2
  Sigma3 : Inport  Port=3
  Sigma4 : Inport  Port=4
  Sigma5 : Inport  Port=5
  Sigma6 : Inport  Port=6
  alpha1 : Inport  Port=7
  alpha2 : Inport  Port=8
  alpha3 : Inport  Port=9
  alpha4 : Inport  Port=10
  alpha5 : Inport  Port=11
  alpha6 : Inport  Port=12
  Cm3 : Inport  Port=13
  Cm4 : Inport  Port=14
  Normal_React : Inport  Port=15
  Caster_Wheel_N°1 : Subsystem
  Caster_Wheel_N°2 : Subsystem
  Caster_Wheel_N°5 : Subsystem
  Caster_Wheel_N°6 : Subsystem
  Demux : Demux  Outputs=6
  Driving_Wheel_N°3 : Subsystem
  Driving_Wheel_N°4 : Subsystem
  F1L : Outport  PortDimensions=1
  F2L : Outport  Port=2  PortDimensions=1
  F3L : Outport  Port=3  PortDimensions=1
  F4L : Outport  Port=4  PortDimensions=1
  F5L : Outport  Port=5  PortDimensions=1
  F6L : Outport  Port=6  PortDimensions=1
  F1T : Outport  Port=7  PortDimensions=1
  F2T : Outport  Port=8  PortDimensions=1
  F3T : Outport  Port=9  PortDimensions=1
  F4T : Outport  Port=10  PortDimensions=1
  F5T : Outport  Port=11  PortDimensions=1
  F6T : Outport  Port=12  PortDimensions=1
  M33 : Outport  Port=13  PortDimensions=1
  M43 : Outport  Port=14  PortDimensions=1
  Thetad_1 : Outport  Port=15  PortDimensions=1
  Thetad_2 : Outport  Port=16  PortDimensions=1
  Thetad_3 : Outport  Port=17  PortDimensions=1
  Thetad_4 : Outport  Port=18  PortDimensions=1
  Thetad_5 : Outport  Port=19  PortDimensions=1
  Thetad_6 : Outport  Port=20  PortDimensions=1
  Phid_1 : Outport  Port=21  PortDimensions=1
  Phid_2 : Outport  Port=22  PortDimensions=1
  Phid_5 : Outport  Port=23  PortDimensions=1
  Phid_6 : Outport  Port=24  PortDimensions=1
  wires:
  Sigma5/1 -> Caster_Wheel_N°5/1(Sigma5)
  Caster_Wheel_N°6/1(F6L) -> F6L/1
  Sigma2/1 -> Caster_Wheel_N°2/1(Sigma2)
  Caster_Wheel_N°6/3(Thetad_6) -> Thetad_6/1
  Caster_Wheel_N°2/1(F2L) -> F2L/1
  Caster_Wheel_N°6/4(Phid_6) -> Phid_6/1
  Caster_Wheel_N°5/3(Thetad_5) -> Thetad_5/1
  alpha1/1 -> Caster_Wheel_N°1/2(alpha1)
  Sigma1/1 -> Caster_Wheel_N°1/1(Sigma1)
  Caster_Wheel_N°1/2(F1T) -> F1T/1
  Caster_Wheel_N°1/4(Phid_1) -> Phid_1/1
  Caster_Wheel_N°5/2(F5T) -> F5T/1
  Caster_Wheel_N°5/4(Phid_5) -> Phid_5/1
  Caster_Wheel_N°5/1(F5L) -> F5L/1
  Caster_Wheel_N°6/2(F6T) -> F6T/1
  Sigma6/1 -> Caster_Wheel_N°6/1(Sigma6)
  alpha6/1 -> Caster_Wheel_N°6/2(alpha6)
  Caster_Wheel_N°2/4(Phid_2) -> Phid_2/1
  alpha5/1 -> Caster_Wheel_N°5/2(alpha5)
  Caster_Wheel_N°2/2(F2T) -> F2T/1
  Caster_Wheel_N°1/1(F1L) -> F1L/1
  alpha2/1 -> Caster_Wheel_N°2/2(alpha2)
  Caster_Wheel_N°2/3(Thetad_2) -> Thetad_2/1
  Caster_Wheel_N°1/3(Thetad_1) -> Thetad_1/1
  alpha4/1 -> Driving_Wheel_N°4/3(alpha4)
  alpha3/1 -> Driving_Wheel_N°3/3(alpha3)
  Driving_Wheel_N°4/2(F4T) -> F4T/1
  Driving_Wheel_N°3/3(M33) -> M33/1
  Driving_Wheel_N°4/4(Thetad_4) -> Thetad_4/1
  Sigma4/1 -> Driving_Wheel_N°4/2(Sigma4)
  Driving_Wheel_N°4/3(M43) -> M43/1
  Sigma3/1 -> Driving_Wheel_N°3/2(Sigma3)
  Driving_Wheel_N°3/1(F3L) -> F3L/1
  Cm3/1 -> Driving_Wheel_N°3/1(Cm3)
  Driving_Wheel_N°3/4(Thetad_3) -> Thetad_3/1
  Driving_Wheel_N°3/2(F3T) -> F3T/1
  Driving_Wheel_N°4/1(F4L) -> F4L/1
  Cm4/1 -> Driving_Wheel_N°4/1(Cm4)
  Normal_React/1 -> Demux/1
  [F13] -> Caster_Wheel_N°1/3(F13)
  [F23] -> Caster_Wheel_N°2/3(F23)
  [F53] -> Caster_Wheel_N°5/3(F53)
  [F63] -> Caster_Wheel_N°6/3(F63)
  [F33] -> Driving_Wheel_N°3/4(F33)
  [F43] -> Driving_Wheel_N°4/4(F43)
  Demux/1 -> [F13]
  Demux/2 -> [F23]
  Demux/3 -> [F33]
  Demux/4 -> [F43]
  Demux/5 -> [F53]
  Demux/6 -> [F63]

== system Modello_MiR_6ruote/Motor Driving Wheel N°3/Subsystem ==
  Thetad_SET : Inport
  Thetad_FB : Inport  Port=2
  iFB : Inport  Port=3
  " " : slpidlib/PID Controller  Controller=PID  Form=Parallel  TimeDomain=Continuous-time  UseExternalTs=off  SampleTime=-1  IntegratorMethod=Forward Euler  FilterMethod=Forward Euler  ControllerParametersSource=internal  P=Kp_v  I=Ki_v  UseKiTs=off  D=0  N=1  UseFilter=on  TunerSelectOption=Transfer Function Based (PID Tuner App)  InitialConditionSource=internal  InitialConditionForIntegrator=0  InitialConditionForFilter=0  DifferentiatorICPrevScaledInput=0  ExternalReset=none  TrackingMode=off  Kt=1  LimitOutput=on  SatLimitsSource=internal  UpperSaturationLimit=iMax  LowerSaturationLimit=-iMax  LinearizeAsGain=on  AntiWindupMode=back-calculation  Kb=1  POutMin=[]  POutMax=[]  IOutMin=[]  IOutMax=[]  DOutMin=[]  DOutMax=[]  NOutMin=[]  NOutMax=[]  SumOutMin=[]  SumOutMax=[]  SaturationOutMin=[]  SaturationOutMax=[]  PParamMin=0  PParamMax=[]  IParamMin=0  IParamMax=[]  DParamMin=0  DParamMax=[]  NParamMin=[]  NParamMax=[]  KbParamMin=[]  KbParamMax=[]  KtParamMin=[]  KtParamMax=[]  KbOutMin=[]  KbOutMax=[]  KtOutMin=[]  KtOutMax=[]  IntegratorOutMin=[]  IntegratorOutMax=[]  FilterOutMin=[]  FilterOutMax=[]  SumI1OutMin=[]  SumI1OutMax=[]  SumI2OutMin=[]  SumI2OutMax=[]  SumI3OutMin=[]  SumI3OutMax=[]  SumI4OutMin=[]  SumI4OutMax=[]  SumDOutMin=[]  SumDOutMax=[]  DifferentiatorOutMin=[]  DifferentiatorOutMax=[]  FilterDiffOutCoefMin=[]  FilterDiffOutCoefMax=[]  ReciprocalOutMin=[]  ReciprocalOutMax=[]  SumDenOutMin=[]  SumDenOutMax=[]  SumNumOutMin=[]  SumNumOutMax=[]  DivideOutMin=[]  DivideOutMax=[]  UdiffTsProdOutMin=[]  UdiffTsProdOutMax=[]  NTsProdOutMin=[]  NTsProdOutMax=[]  UintegralTsProdOutMin=[]  UintegralTsProdOutMax=[]  UngainTsProdOutMin=[]  UngainTsProdOutMax=[]  IntegratorContinuousStateAttributes=''  IntegratorStateMustResolveToSignalObject=off  IntegratorRTWStateStorageClass=Auto  FilterContinuousStateAttributes=''  FilterStateMustResolveToSignalObject=off  FilterRTWStateStorageClass=Auto  ParallelPVariant=InternalParameters  IdealPVariant=Disabled  IVariant=InternalParameters  DVariant=InternalParameters  IntegratorVariant=Continuous  SatVariant=Enabled  AWVariant=BackCalculation  PCopyVariant=Disabled  TRVariant=Disabled  FdbkBlocksVariant=Forward  IdealPFdbkVariant=Disabled  SatFdbkVariant=Disabled  DerivativeFilterVariant=ContFilter  NVariant=InternalParameters  NCopyVariant=Disabled  FilterICVariant=InternalICsFilter  IntegratorICVariant=InternalICs  ExternalResetVariant=Disabled  TRSumVariant=Passthrough  SumFdbkVariant=Disabled  SumVariant=Sum_PID  TsampFilterVariant=InternalTs  TsampNgainVariant=Passthrough  TsampIntegralVariant=Passthrough  ExternalSaturationOutDataTypeStr=Inherit: Same as second input  aMode=0
  PID Controller1 : slpidlib/PID Controller  Controller=PID  Form=Parallel  TimeDomain=Continuous-time  UseExternalTs=off  SampleTime=-1  IntegratorMethod=Forward Euler  FilterMethod=Forward Euler  ControllerParametersSource=internal  P=Kp_i  I=Ki_i  UseKiTs=off  D=0  N=100  UseFilter=on  TunerSelectOption=Transfer Function Based (PID Tuner App)  InitialConditionSource=internal  InitialConditionForIntegrator=0  InitialConditionForFilter=0  DifferentiatorICPrevScaledInput=0  ExternalReset=none  TrackingMode=off  Kt=1  LimitOutput=on  SatLimitsSource=internal  UpperSaturationLimit=VaMax  LowerSaturationLimit=-VaMax  LinearizeAsGain=on  AntiWindupMode=back-calculation  Kb=1  POutMin=[]  POutMax=[]  IOutMin=[]  IOutMax=[]  DOutMin=[]  DOutMax=[]  NOutMin=[]  NOutMax=[]  SumOutMin=[]  SumOutMax=[]  SaturationOutMin=[]  SaturationOutMax=[]  PParamMin=[]  PParamMax=[]  IParamMin=[]  IParamMax=[]  DParamMin=[]  DParamMax=[]  NParamMin=[]  NParamMax=[]  KbParamMin=[]  KbParamMax=[]  KtParamMin=[]  KtParamMax=[]  KbOutMin=[]  KbOutMax=[]  KtOutMin=[]  KtOutMax=[]  IntegratorOutMin=[]  IntegratorOutMax=[]  FilterOutMin=[]  FilterOutMax=[]  SumI1OutMin=[]  SumI1OutMax=[]  SumI2OutMin=[]  SumI2OutMax=[]  SumI3OutMin=[]  SumI3OutMax=[]  SumI4OutMin=[]  SumI4OutMax=[]  SumDOutMin=[]  SumDOutMax=[]  DifferentiatorOutMin=[]  DifferentiatorOutMax=[]  FilterDiffOutCoefMin=[]  FilterDiffOutCoefMax=[]  ReciprocalOutMin=[]  ReciprocalOutMax=[]  SumDenOutMin=[]  SumDenOutMax=[]  SumNumOutMin=[]  SumNumOutMax=[]  DivideOutMin=[]  DivideOutMax=[]  UdiffTsProdOutMin=[]  UdiffTsProdOutMax=[]  NTsProdOutMin=[]  NTsProdOutMax=[]  UintegralTsProdOutMin=[]  UintegralTsProdOutMax=[]  UngainTsProdOutMin=[]  UngainTsProdOutMax=[]  IntegratorContinuousStateAttributes=''  IntegratorStateMustResolveToSignalObject=off  IntegratorRTWStateStorageClass=Auto  FilterContinuousStateAttributes=''  FilterStateMustResolveToSignalObject=off  FilterRTWStateStorageClass=Auto  ParallelPVariant=InternalParameters  IdealPVariant=Disabled  IVariant=InternalParameters  DVariant=InternalParameters  IntegratorVariant=Continuous  SatVariant=Enabled  AWVariant=BackCalculation  PCopyVariant=Disabled  TRVariant=Disabled  FdbkBlocksVariant=Forward  IdealPFdbkVariant=Disabled  SatFdbkVariant=Disabled  DerivativeFilterVariant=ContFilter  NVariant=InternalParameters  NCopyVariant=Disabled  FilterICVariant=InternalICsFilter  IntegratorICVariant=InternalICs  ExternalResetVariant=Disabled  TRSumVariant=Passthrough  SumFdbkVariant=Disabled  SumVariant=Sum_PID  TsampFilterVariant=InternalTs  TsampNgainVariant=Passthrough  TsampIntegralVariant=Passthrough  ExternalSaturationOutDataTypeStr=Inherit: Same as second input  aMode=0
  Scope : Scope
  Scope1 : Scope
  Scope2 : Scope
  Scope3 : Scope  NumInputPorts=2
  Sum1 : Sum  Inputs=|+-
  Sum2 : Sum  Inputs=|+-
  VaRif : Outport  VectorParamsAs1DForOutWhenUnconnected=off
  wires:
  Thetad_FB/1 -> Scope3/2, Sum1/2
  " "/1 -> Scope2/1, Sum2/1
  PID Controller1/1 -> Scope1/1, VaRif/1
  iFB/1 -> Sum2/2
  Thetad_SET/1 -> Scope3/1, Sum1/1
  Sum1/1 -> Scope/1, " "/1
  Sum2/1 -> PID Controller1/1

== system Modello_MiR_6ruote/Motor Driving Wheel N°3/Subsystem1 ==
  VaRif : Inport
  Thetad_FB : Inport  Port=2
  Add : Sum  Inputs=+--
  Gain : Gain  Gain=rap_rid
  Gain1 : Gain  Gain=1/L
  Gain2 : Gain  Gain=Kc
  Gain3 : Gain  Gain=R
  Gain4 : Gain  Gain=Kc
  Integrator : Integrator
  Scope : Scope
  Scope1 : Scope
  Torque Cm : Outport  VectorParamsAs1DForOutWhenUnconnected=off
  iFB : Outport  Port=2  VectorParamsAs1DForOutWhenUnconnected=off
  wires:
  VaRif/1 -> Add/1
  Add/1 -> Gain1/1
  Gain1/1 -> Integrator/1
  Integrator/1 -> Gain4/1, iFB/1, Gain3/1
  Gain3/1 -> Add/3
  Gain4/1 -> Scope1/1, Gain/1
  Thetad_FB/1 -> Gain2/1, Scope/1
  Gain2/1 -> Add/2
  Gain/1 -> Torque Cm/1

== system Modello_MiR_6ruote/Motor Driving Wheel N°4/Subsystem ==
  Thetad_SET : Inport
  Thetad_FB : Inport  Port=2
  iFB : Inport  Port=3
  " " : slpidlib/PID Controller  Controller=PID  Form=Parallel  TimeDomain=Continuous-time  UseExternalTs=off  SampleTime=-1  IntegratorMethod=Forward Euler  FilterMethod=Forward Euler  ControllerParametersSource=internal  P=Kp_v  I=Ki_v  UseKiTs=off  D=0  N=1  UseFilter=on  TunerSelectOption=Transfer Function Based (PID Tuner App)  InitialConditionSource=internal  InitialConditionForIntegrator=0  InitialConditionForFilter=0  DifferentiatorICPrevScaledInput=0  ExternalReset=none  TrackingMode=off  Kt=1  LimitOutput=on  SatLimitsSource=internal  UpperSaturationLimit=iMax  LowerSaturationLimit=-iMax  LinearizeAsGain=on  AntiWindupMode=back-calculation  Kb=1  POutMin=[]  POutMax=[]  IOutMin=[]  IOutMax=[]  DOutMin=[]  DOutMax=[]  NOutMin=[]  NOutMax=[]  SumOutMin=[]  SumOutMax=[]  SaturationOutMin=[]  SaturationOutMax=[]  PParamMin=0  PParamMax=[]  IParamMin=0  IParamMax=[]  DParamMin=0  DParamMax=[]  NParamMin=[]  NParamMax=[]  KbParamMin=[]  KbParamMax=[]  KtParamMin=[]  KtParamMax=[]  KbOutMin=[]  KbOutMax=[]  KtOutMin=[]  KtOutMax=[]  IntegratorOutMin=[]  IntegratorOutMax=[]  FilterOutMin=[]  FilterOutMax=[]  SumI1OutMin=[]  SumI1OutMax=[]  SumI2OutMin=[]  SumI2OutMax=[]  SumI3OutMin=[]  SumI3OutMax=[]  SumI4OutMin=[]  SumI4OutMax=[]  SumDOutMin=[]  SumDOutMax=[]  DifferentiatorOutMin=[]  DifferentiatorOutMax=[]  FilterDiffOutCoefMin=[]  FilterDiffOutCoefMax=[]  ReciprocalOutMin=[]  ReciprocalOutMax=[]  SumDenOutMin=[]  SumDenOutMax=[]  SumNumOutMin=[]  SumNumOutMax=[]  DivideOutMin=[]  DivideOutMax=[]  UdiffTsProdOutMin=[]  UdiffTsProdOutMax=[]  NTsProdOutMin=[]  NTsProdOutMax=[]  UintegralTsProdOutMin=[]  UintegralTsProdOutMax=[]  UngainTsProdOutMin=[]  UngainTsProdOutMax=[]  IntegratorContinuousStateAttributes=''  IntegratorStateMustResolveToSignalObject=off  IntegratorRTWStateStorageClass=Auto  FilterContinuousStateAttributes=''  FilterStateMustResolveToSignalObject=off  FilterRTWStateStorageClass=Auto  ParallelPVariant=InternalParameters  IdealPVariant=Disabled  IVariant=InternalParameters  DVariant=InternalParameters  IntegratorVariant=Continuous  SatVariant=Enabled  AWVariant=BackCalculation  PCopyVariant=Disabled  TRVariant=Disabled  FdbkBlocksVariant=Forward  IdealPFdbkVariant=Disabled  SatFdbkVariant=Disabled  DerivativeFilterVariant=ContFilter  NVariant=InternalParameters  NCopyVariant=Disabled  FilterICVariant=InternalICsFilter  IntegratorICVariant=InternalICs  ExternalResetVariant=Disabled  TRSumVariant=Passthrough  SumFdbkVariant=Disabled  SumVariant=Sum_PID  TsampFilterVariant=InternalTs  TsampNgainVariant=Passthrough  TsampIntegralVariant=Passthrough  ExternalSaturationOutDataTypeStr=Inherit: Same as second input  aMode=0
  PID Controller1 : slpidlib/PID Controller  Controller=PID  Form=Parallel  TimeDomain=Continuous-time  UseExternalTs=off  SampleTime=-1  IntegratorMethod=Forward Euler  FilterMethod=Forward Euler  ControllerParametersSource=internal  P=Kp_i  I=Ki_i  UseKiTs=off  D=0  N=100  UseFilter=on  TunerSelectOption=Transfer Function Based (PID Tuner App)  InitialConditionSource=internal  InitialConditionForIntegrator=0  InitialConditionForFilter=0  DifferentiatorICPrevScaledInput=0  ExternalReset=none  TrackingMode=off  Kt=1  LimitOutput=on  SatLimitsSource=internal  UpperSaturationLimit=VaMax  LowerSaturationLimit=-VaMax  LinearizeAsGain=on  AntiWindupMode=back-calculation  Kb=1  POutMin=[]  POutMax=[]  IOutMin=[]  IOutMax=[]  DOutMin=[]  DOutMax=[]  NOutMin=[]  NOutMax=[]  SumOutMin=[]  SumOutMax=[]  SaturationOutMin=[]  SaturationOutMax=[]  PParamMin=[]  PParamMax=[]  IParamMin=[]  IParamMax=[]  DParamMin=[]  DParamMax=[]  NParamMin=[]  NParamMax=[]  KbParamMin=[]  KbParamMax=[]  KtParamMin=[]  KtParamMax=[]  KbOutMin=[]  KbOutMax=[]  KtOutMin=[]  KtOutMax=[]  IntegratorOutMin=[]  IntegratorOutMax=[]  FilterOutMin=[]  FilterOutMax=[]  SumI1OutMin=[]  SumI1OutMax=[]  SumI2OutMin=[]  SumI2OutMax=[]  SumI3OutMin=[]  SumI3OutMax=[]  SumI4OutMin=[]  SumI4OutMax=[]  SumDOutMin=[]  SumDOutMax=[]  DifferentiatorOutMin=[]  DifferentiatorOutMax=[]  FilterDiffOutCoefMin=[]  FilterDiffOutCoefMax=[]  ReciprocalOutMin=[]  ReciprocalOutMax=[]  SumDenOutMin=[]  SumDenOutMax=[]  SumNumOutMin=[]  SumNumOutMax=[]  DivideOutMin=[]  DivideOutMax=[]  UdiffTsProdOutMin=[]  UdiffTsProdOutMax=[]  NTsProdOutMin=[]  NTsProdOutMax=[]  UintegralTsProdOutMin=[]  UintegralTsProdOutMax=[]  UngainTsProdOutMin=[]  UngainTsProdOutMax=[]  IntegratorContinuousStateAttributes=''  IntegratorStateMustResolveToSignalObject=off  IntegratorRTWStateStorageClass=Auto  FilterContinuousStateAttributes=''  FilterStateMustResolveToSignalObject=off  FilterRTWStateStorageClass=Auto  ParallelPVariant=InternalParameters  IdealPVariant=Disabled  IVariant=InternalParameters  DVariant=InternalParameters  IntegratorVariant=Continuous  SatVariant=Enabled  AWVariant=BackCalculation  PCopyVariant=Disabled  TRVariant=Disabled  FdbkBlocksVariant=Forward  IdealPFdbkVariant=Disabled  SatFdbkVariant=Disabled  DerivativeFilterVariant=ContFilter  NVariant=InternalParameters  NCopyVariant=Disabled  FilterICVariant=InternalICsFilter  IntegratorICVariant=InternalICs  ExternalResetVariant=Disabled  TRSumVariant=Passthrough  SumFdbkVariant=Disabled  SumVariant=Sum_PID  TsampFilterVariant=InternalTs  TsampNgainVariant=Passthrough  TsampIntegralVariant=Passthrough  ExternalSaturationOutDataTypeStr=Inherit: Same as second input  aMode=0
  Scope : Scope  NumInputPorts=2
  Sum1 : Sum  Inputs=|+-
  Sum2 : Sum  Inputs=|+-
  VaRif : Outport  VectorParamsAs1DForOutWhenUnconnected=off
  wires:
  Thetad_FB/1 -> Scope/2, Sum1/2
  " "/1 -> Sum2/1
  PID Controller1/1 -> VaRif/1
  iFB/1 -> Sum2/2
  Thetad_SET/1 -> Scope/1, Sum1/1
  Sum1/1 -> " "/1
  Sum2/1 -> PID Controller1/1

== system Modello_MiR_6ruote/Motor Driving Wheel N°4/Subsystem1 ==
  VaRif : Inport
  Thetad_FB : Inport  Port=2
  Add : Sum  Inputs=+--
  Gain : Gain  Gain=rap_rid
  Gain1 : Gain  Gain=1/L
  Gain2 : Gain  Gain=Kc
  Gain3 : Gain  Gain=R
  Gain4 : Gain  Gain=Kc
  Integrator : Integrator
  Scope : Scope
  Scope1 : Scope
  Torque Cm : Outport  VectorParamsAs1DForOutWhenUnconnected=off
  iFB : Outport  Port=2  VectorParamsAs1DForOutWhenUnconnected=off
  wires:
  VaRif/1 -> Add/1
  Add/1 -> Gain1/1
  Gain1/1 -> Integrator/1
  Integrator/1 -> Gain4/1, Gain3/1, iFB/1
  Gain3/1 -> Add/3
  Thetad_FB/1 -> Gain2/1, Scope/1
  Gain2/1 -> Add/2
  Gain4/1 -> Gain/1
  Gain/1 -> Scope1/1, Torque Cm/1

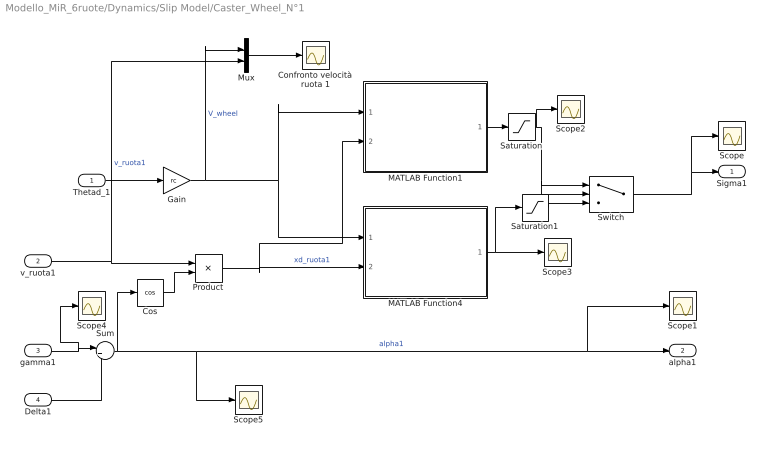
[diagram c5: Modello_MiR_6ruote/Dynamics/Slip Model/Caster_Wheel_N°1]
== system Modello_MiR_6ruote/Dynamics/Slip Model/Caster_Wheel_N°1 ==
  Thetad_1 : Inport
  v_ruota1 : Inport  Port=2
  gamma1 : Inport  Port=3
  Delta1 : Inport  Port=4
  Confronto velocità ruota 1 : Scope
  Cos : Trigonometry  Operator=cos
  Gain : Gain  Gain=rc
  MATLAB Function1 : MATLAB Function  TreatAsAtomicUnit=on
  MATLAB Function4 : MATLAB Function  TreatAsAtomicUnit=on
  Mux : Mux  Inputs=2
  Product : Product
  Saturation : Saturate  UpperLimit=1  LowerLimit=-1
  Saturation1 : Saturate  UpperLimit=1  LowerLimit=-1
  Scope{,1..5} (6 alike) : Scope
  Sum : Sum  Inputs=|+-
  Switch : Switch
  Sigma1 : Outport
  alpha1 : Outport  Port=2
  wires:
  Thetad_1/1 -> Gain/1
  Gain/1 -> Mux/1, MATLAB Function4/1(v_wheel), MATLAB Function1/1(v_wheel)  "V_wheel"
  Switch/1 -> Scope/1, Sigma1/1
  MATLAB Function1/1(Fc_pos_out) -> Saturation/1
  MATLAB Function4/1(Fc_neg_out) -> Saturation1/1, Scope3/1
  Product/1 -> MATLAB Function1/2(xd_ruota1), MATLAB Function4/2(xd_ruota1)  "xd_ruota1"
  v_ruota1/1 -> Mux/2, Product/1  "v_ruota1"
  Cos/1 -> Product/2
  Delta1/1 -> Sum/2
  Sum/1 -> Cos/1, Scope1/1, alpha1/1, Scope5/1  "alpha1"
  Mux/1 -> Confronto velocità ruota 1/1
  Saturation/1 -> Scope2/1, Switch/1, Switch/2
  Saturation1/1 -> Switch/3
  gamma1/1 -> Scope4/1, Sum/1
